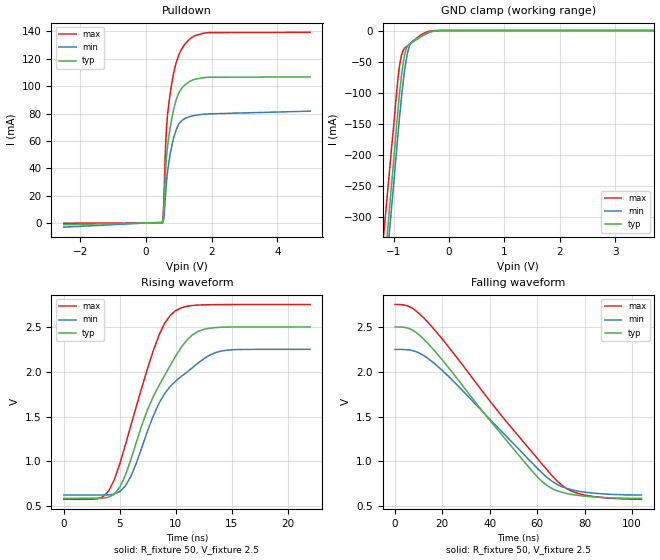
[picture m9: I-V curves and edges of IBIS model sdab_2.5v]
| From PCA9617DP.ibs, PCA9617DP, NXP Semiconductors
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[Model]   sdab_2.5v
Model_type Open_drain
Vref=2.500E+00
Rref=1.350E+03
Cref=5.000E-11
Vmeas=1.250E+00
C_comp   8.050E-13   7.840E-13   8.260E-13
[Voltage Range]   2.500E+00   2.250E+00   2.750E+00
[POWER Clamp Reference]   2.500E+00   2.250E+00   2.750E+00
[GND Clamp Reference]   0.000E+00   0.000E+00   0.000E+00
[Pullup Reference]   2.500E+00   2.250E+00   2.750E+00
[Pulldown Reference]   0.000E+00   0.000E+00   0.000E+00
[Temperature Range]   25   85   -40
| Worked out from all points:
|   slope of the pulldown table from 0 to 0.375 V, typ, clamps not added: 2.78 kohm
|   GND clamp passes 1 mA (typ) near -0.29 V on its own axis
|   rising waveform, R_fixture 50, V_fixture 2.5: 20-80 % time 3.88ns typ, 3.9ns min, 3.13ns max; typ from 0.589 V to 2.5 V
|   falling waveform, R_fixture 50, V_fixture 2.5: 20-80 % time 35ns typ, 35.6ns min, 39.3ns max; typ from 2.5 V to 0.589 V
[GND Clamp]
-2.5V     -1.758A    -1.768A    -1.615A
-1.02V    -228.4mA   -265.7mA   -170.8mA
-940mV    -145.4mA   -184.3mA   -91.91mA
-900mV    -106.4mA   -144.6mA   -60.01mA
-880mV    -88.82mA   -125.8mA   -48.49mA
-820mV    -47.24mA   -75.88mA   -30.76mA
-760mV    -26.77mA   -40.13mA   -25.19mA
-720mV    -22.18mA   -25.66mA   -22.46mA
-680mV    -19.76mA   -18.42mA   -19.41mA
-460mV    -6.779mA   -7.485mA   -4.555mA
-160mV    0A         0A         0A
5V        0A         0A         0A
[Pulldown]
-2.5V     -1.23mA    -3.035mA   -180.8uA
500mV     180.1uA    83.86uA    483.3uA
540mV     6.774mA    2.075mA    12.07mA
600mV     37.73mA    21.12mA    56.16mA
620mV     45.59mA    27.77mA    66.31mA
660mV     56.17mA    37.54mA    79.11mA
760mV     72.56mA    52.83mA    97.83mA
860mV     84.46mA    63.4mA     111.1mA
1V        94.92mA    72.15mA    122.7mA
1.34V     103.5mA    77.79mA    134.5mA
1.92V     106.5mA    79.75mA    139.1mA
5V        106.7mA    81.72mA    139.3mA
[Rising Waveform]
R_fixture = 50
V_fixture = 2.5
V_fixture_min = 2.25
V_fixture_max = 2.75
0s        588.8mV    626.4mV    578.2mV
4ns       601.3mV    627.8mV    669.4mV
5ns       712.5mV    664.2mV    971.6mV
6ns       1.024V     835mV      1.405V
7.5ns     1.583V     1.346V     2.044V
8.5ns     1.846V     1.647V     2.407V
10ns      2.176V     1.897V     2.682V
12.5ns    2.472V     2.145V     2.746V
14.5ns    2.498V     2.24V      2.749V
22ns      2.5V       2.25V      2.75V
[Falling Waveform]
R_fixture = 50
V_fixture = 2.5
V_fixture_min = 2.25
V_fixture_max = 2.75
0s        2.5V       2.25V      2.75V
7.5ns     2.463V     2.235V     2.705V
16.5ns    2.241V     2.096V     2.474V
26ns      1.932V     1.859V     2.163V
54.5ns    998.6mV    1.075V     1.209V
64ns      736.1mV    826.2mV    912.1mV
70.5ns    656.4mV    718.7mV    734.5mV
76.5ns    624.6mV    672.9mV    650.5mV
86.5ns    600.5mV    641.4mV    600.8mV
104ns     588.8mV    626.4mV    578.2mV
[Ramp]
dV/dt_r   1.1467E+00/3.8660E-09   9.7413E-01/3.8790E-09   1.3031E+00/3.1160E-09
dV/dt_f   1.1467E+00/3.4955E-08   9.7413E-01/3.5560E-08   1.3031E+00/3.9316E-08
R_load = 50
